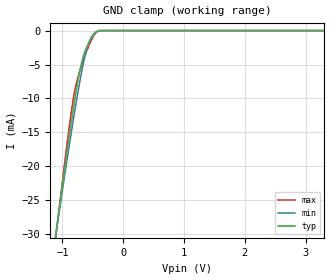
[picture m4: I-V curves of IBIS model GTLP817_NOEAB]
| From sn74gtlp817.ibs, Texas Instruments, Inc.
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[Model]   GTLP817_NOEAB
Model_type  Input
Vinl=0.8
Vinh=2.0
| variable   typ   min   max
C_comp   2.85pF   2.04pF   3.97pF
[Temperature Range]   40   100   -40
| Ambient temperature   25   85   -40
[Voltage range]   3.3   3.15   3.45
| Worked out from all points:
|   GND clamp passes 1 mA (typ) near -0.51 V on its own axis
[GND Clamp]
| GTLP817_NOEAB
|   Voltage   I(typ)   I(min)   I(max)
-5.5V     -349.9mA   -322.6mA   -391.6mA
-1.135V   -31.72mA   -31.74mA   -32.32mA
-1.095V   -29.05mA   -29.29mA   -29.29mA
-900mV    -16.41mA   -17.67mA   -15.06mA
-835mV    -12.45mA   -13.97mA   -10.86mA
-790mV    -9.847mA   -11.49mA   -8.536mA
-690mV    -4.948mA   -6.385mA   -5.276mA
-605mV    -2.528mA   -2.9mA     -3.115mA
-540mV    -1.394mA   -1.229mA   -1.719mA
-450mV    -300.1uA   -191.4uA   -334.8uA
-360mV    -3.423uA   -9.411uA   -3.546uA
3.3V      169.1pA    605.3pA    1.317nA
